FUNCTION_BLOCK Example23_holdfor //4x3 flyways 4 xbots - HoldForPMCState, HoldForXbot(s)Idle, HoldForXbot(s)State
VAR_INPUT
	Execute : BOOL;
END_VAR
VAR_OUTPUT
	Done : BOOL;
END_VAR
VAR_IN_OUT
	PM_Controller : PMControllerType;	// the planar motor controller to use
END_VAR
VAR
	PMC_Reboot1 : PMC_Reboot;
	PMC_HoldForPMCState1 : PMC_HoldForPMCState;
	Delay1 : Delay;
	PMC_ActivateXbots1 : PMC_ActivateXbots;
	PMC_HoldForXbotIdle1 : PMC_HoldForXbotIdle;
	xbotID_array78 : ARRAY[0..77] OF USINT;
	posX_array78 : ARRAY[0..77] OF REAL;
	posY_array78 : ARRAY[0..77] OF REAL;
	PMC_AutoDrivingMotionVelocity1 : PMC_AutoDrivingMotionVelocity;
	PMC_HoldForXbotState1 : PMC_HoldForXbotState;
	PMC_XYMotion1 : PMC_XYMotion;
	PMC_XYMotion2 : PMC_XYMotion;
	PMC_XYMotion3 : PMC_XYMotion;
	PMC_XYMotion4 : PMC_XYMotion;
	PMC_HoldForXbotsIdle1 : PMC_HoldForXbotsIdle;
	PMC_XYMotion5 : PMC_XYMotion;
	PMC_LevitationCtrl1 : PMC_LevitationCtrl;
	state_array78 : ARRAY[0..77] OF USINT;
	PMC_HoldForXbotsState1 : PMC_HoldForXbotsState;
END_VAR

//4x3 flyways 4 xbots - HoldForPMCState, HoldForXbot(s)Idle, HoldForXbot(s)State

//reboot PMC
PMC_Reboot1(Execute := Execute,PM_Controller := PM_Controller);

//hold until PMC is done rebooting and is inactive
PMC_HoldForPMCState1(Execute := PMC_Reboot1.Ack,State := 1,PM_Controller := PM_Controller);

Delay1(Execute := PMC_HoldForPMCState1.Done,Cycles := 5000);

//activate xbots
PMC_ActivateXbots1(Execute := Delay1.Done,PM_Controller := PM_Controller);

//hold until xbot 4 is idle
PMC_HoldForXbotIdle1(Execute := PMC_ActivateXbots1.Ack,XbotID := 4,PM_Controller := PM_Controller);

//move all xbots to bottom of flyways
xbotID_array78[0] := 1;xbotID_array78[1] := 2;xbotID_array78[2] := 3;xbotID_array78[3] := 4;
posX_array78[0] := 0.06;posX_array78[1] := 0.3;posX_array78[2] := 0.54;posX_array78[3] := 0.78;
posY_array78[0] := 0.06;posY_array78[1] := 0.06;posY_array78[2] := 0.06;posY_array78[3] := 0.06;
PMC_AutoDrivingMotionVelocity1(Execute := PMC_HoldForXbotIdle1.Done,nXbots := 4,RoutingType := 0,ZoneID := 0,XbotID := xbotID_array78,PosX := posX_array78,PosY := posY_array78,MaxVel := 1,MaxAcc := 10,PM_Controller := PM_Controller);

//hold until xbot 2 is idle
PMC_HoldForXbotState1(Execute := PMC_AutoDrivingMotionVelocity1.Ack,XbotID := 2,State := 3,PM_Controller := PM_Controller);

//move all xbots to the bottom of flyways at different speeds
PMC_XYMotion1(Execute := PMC_HoldForXbotState1.Done,cmdLB := 7,XbotID := 1,Mode := 0,Type_ := 0,PosX := 0.06,PosY := 0.66,EndVel := 0,MaxVel := 1,MaxAcc := 10,PM_Controller := PM_Controller);
PMC_XYMotion2(Execute := PMC_XYMotion1.Ack,cmdLB := 8,XbotID := 2,Mode := 0,Type_ := 0,PosX := 0.3,PosY := 0.66,EndVel := 0,MaxVel := 2,MaxAcc := 20,PM_Controller := PM_Controller);
PMC_XYMotion3(Execute := PMC_XYMotion2.Ack,cmdLB := 9,XbotID := 3,Mode := 0,Type_ := 0,PosX := 0.54,PosY := 0.66,EndVel := 0,MaxVel := 0.5,MaxAcc := 5,PM_Controller := PM_Controller);
PMC_XYMotion4(Execute := PMC_XYMotion3.Ack,cmdLB := 10,XbotID := 4,Mode := 0,Type_ := 0,PosX := 0.78,PosY := 0.66,EndVel := 0,MaxVel := 2,MaxAcc := 0.1,PM_Controller := PM_Controller);

//hold until all xbots are idle
xbotID_array78[0] := 1;xbotID_array78[1] := 2;xbotID_array78[2] := 3;xbotID_array78[3] := 4;
PMC_HoldForXbotsIdle1(Execute := PMC_XYMotion4.Ack,nXbots := 4,XbotID := xbotID_array78,PM_Controller := PM_Controller);

//move xbot 1 to bottom of flyway, land xbot 4
PMC_XYMotion5(Execute := PMC_HoldForXbotsIdle1.Done,cmdLB := 12,XbotID := 1,Mode := 0,Type_ := 0,PosX := 0.06,PosY := 0.06,EndVel := 0,MaxVel := 1,MaxAcc := 10,PM_Controller := PM_Controller);
PMC_LevitationCtrl1(Execute := PMC_XYMotion5.Ack,XbotID := 4,Level := 0,Speed := 0,LandedZForce := 0,PM_Controller := PM_Controller);

//hold until xbot 4 is landed and all other xbots are idle
xbotID_array78[0] := 1;xbotID_array78[1] := 2;xbotID_array78[2] := 3;xbotID_array78[3] := 4;
state_array78[0] := 3;state_array78[1] := 3;state_array78[2] := 3;state_array78[3] := 2;
PMC_HoldForXbotsState1(Execute := PMC_LevitationCtrl1.Ack,nXbots := 4,XbotID := xbotID_array78,States := state_array78,PM_Controller := PM_Controller);

Done := PMC_HoldForXbotsState1.Done;

END_FUNCTION_BLOCK
